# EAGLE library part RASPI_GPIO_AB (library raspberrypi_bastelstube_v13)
Only the 2x13 header connector, nothing else
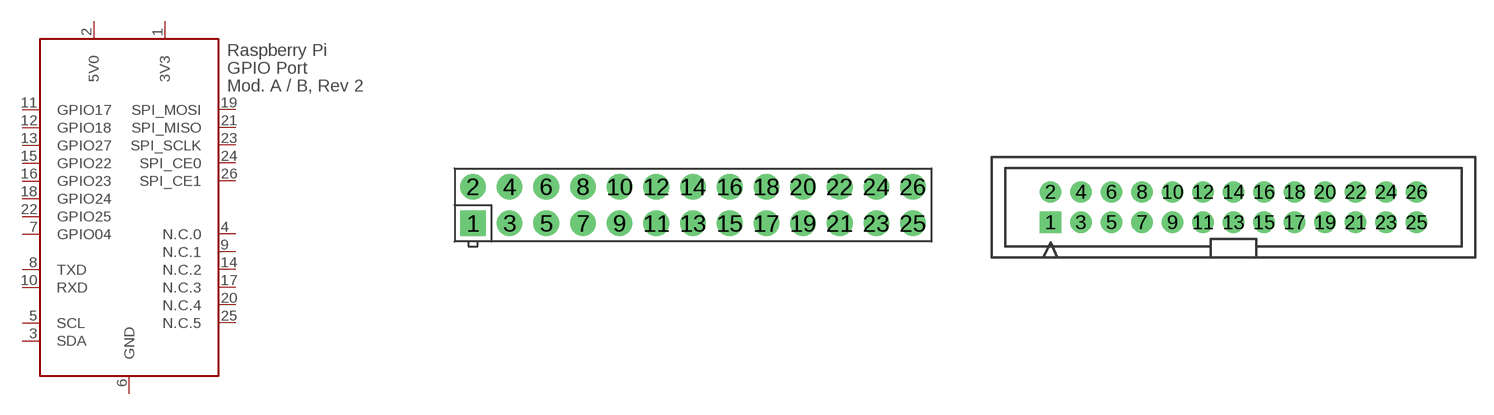
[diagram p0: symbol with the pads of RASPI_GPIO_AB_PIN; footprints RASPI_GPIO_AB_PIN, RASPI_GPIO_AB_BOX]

Designator prefix X

## RASPI_GPIO_AB_PIN  [RASPI_GPIO_AB_PIN]
1  3V3  pwr
2  5V0  pwr
3  SDA
4  N.C.0  nc
5  SCL
6  GND  pwr
7  GPIO04
8  TXD
9  N.C.1  nc
10  RXD
11  GPIO17
12  GPIO18
13  GPIO27
14  N.C.2  nc
15  GPIO22
16  GPIO23
17  N.C.3  nc
18  GPIO24
19  SPI_MOSI
20  N.C.4  nc
21  SPI_MISO
22  GPIO25
23  SPI_SCLK
24  SPI_CE0
25  N.C.5  nc
26  SPI_CE1

## RASPI_GPIO_AB_BOX  [RASPI_GPIO_AB_BOX]
Pads as for RASPI_GPIO_AB_PIN

## Footprint RASPI_GPIO_AB_PIN (pad centres in mm)
26-pin connector for Raspberry Pi GPIO just the two rows of pins
drill 1 pad 1.778 square: 1 -15.24,-1.27
drill 1 pad 1.778: 2 -15.24,1.27; 3 -12.7,-1.27; 4 -12.7,1.27; 5 -10.16,-1.27; 6 -10.16,1.27; 7 -7.62,-1.27; 8 -7.62,1.27; 9 -5.08,-1.27; 10 -5.08,1.27; 11 -2.54,-1.27; 12 -2.54,1.27; 13 0,-1.27; 14 0,1.27; 15 2.54,-1.27; 16 2.54,1.27; 17 5.08,-1.27; 18 5.08,1.27; 19 7.62,-1.27; 20 7.62,1.27; 21 10.16,-1.27; 22 10.16,1.27; 23 12.7,-1.27; 24 12.7,1.27; 25 15.24,-1.27; 26 15.24,1.27

## Footprint RASPI_GPIO_AB_BOX (pad centres in mm)
26-pin box header for Raspberry Pi GPIO for use with flat ribbon cables
drill 1 pad 1.778 square: 1 -15.24,-1.27
drill 1 pad 1.778: 2 -15.24,1.27; 3 -12.7,-1.27; 4 -12.7,1.27; 5 -10.16,-1.27; 6 -10.16,1.27; 7 -7.62,-1.27; 8 -7.62,1.27; 9 -5.08,-1.27; 10 -5.08,1.27; 11 -2.54,-1.27; 12 -2.54,1.27; 13 0,-1.27; 14 0,1.27; 15 2.54,-1.27; 16 2.54,1.27; 17 5.08,-1.27; 18 5.08,1.27; 19 7.62,-1.27; 20 7.62,1.27; 21 10.16,-1.27; 22 10.16,1.27; 23 12.7,-1.27; 24 12.7,1.27; 25 15.24,-1.27; 26 15.24,1.27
